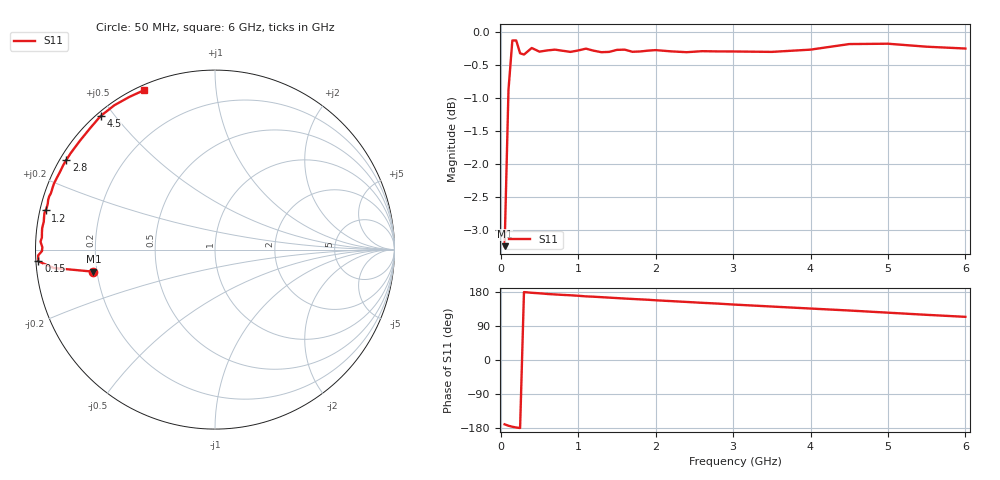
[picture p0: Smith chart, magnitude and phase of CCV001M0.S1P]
! Infineon Technologies  Discrete & RF Semiconductors
! BBY57-02W
! Si Tuning Diode in SCD-80
! VR = 0
! S-Parameters:  June  2000
# GHz  S  MA  R  50
!  f  S11
! GHz  MAG  ANG
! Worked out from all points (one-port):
!   34 points, 50 MHz to 6 GHz, reference 50 ohm
!   lowest |S11| = -3.2 dB at 50 MHz (marker M1), VSWR 5.42, Z = 9.3 - j4.35 ohm
!   |S11| at or under -10 dB: nowhere
!   S11 on the Smith chart (normalised r, x): 50 MHz: 0.19, -0.09; 150 MHz: 0.01, -0.03; 1.2 GHz: 0.02, +0.11; 2.8 GHz: 0.02, +0.28; 4.5 GHz: 0.01, +0.46; 6 GHz: 0.02, +0.65
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0.05  0.6883 -169.7
0.1  0.9045 -173.5
0.15  0.986 -176.2
0.2  0.986 -178.1
0.25  0.9642 -179.5
0.3  0.962 179.2
0.4  0.9731 177.4
0.5  0.9669 176.0
0.6  0.969 174.3
0.8  0.9684 171.8
0.9  0.9665 170.8
1  0.9689 169.5
1.1  0.972 167.9
1.2  0.9685 167.0
1.6  0.9703 162.2
1.7  0.9667 161.1
1.9  0.9686 159.0
2  0.9695 157.6
2.4  0.966 153.2
2.6  0.9677 150.9
2.8  0.9673 148.9
3  0.9672 146.4
3.5  0.9665 141.1
4  0.9703 135.8
4.5  0.9798 130.6
5  0.9804 124.9
5.5  0.9753 119.2
6  0.9722 113.9
